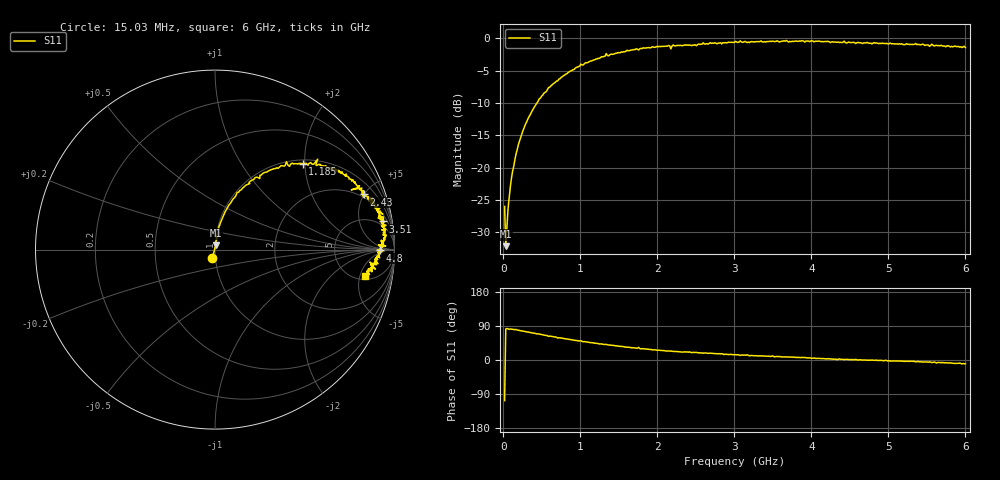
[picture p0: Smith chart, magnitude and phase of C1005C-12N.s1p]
!	Network	Analyzer	HP8753E.07.74:	Oct	30	2002	Serial	No.	JP38451487
!	Hewlett-Packard
!	7	Sep	2009	8:43:02
!	Frequency	S11
#	HZ	S	RI	R	50
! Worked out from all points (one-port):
!   400 points, 15.03 MHz to 6 GHz, reference 50 ohm
!   lowest |S11| = -32.1 dB at 30.03 MHz (marker M1), VSWR 1.05, Z = 50.3 + j2.47 ohm
!   |S11| at or under -10 dB: start of sweep to 435.5 MHz
!   S11 on the Smith chart (normalised r, x): 15.03 MHz: 0.97, -0.09; 1.185 GHz: 1.09, +1.95; 2.43 GHz: 1.77, +4.97; 3.51 GHz: 4, +11; 4.8 GHz: 23, -1; 6 GHz: 5.85, -6.14
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1.502992e7  -0.0148 -0.048
3.002985e7  0.0036 0.0245
6.00297e7  0.00645 0.048
1.050295e8  0.0127 0.0827
1.650292e8  0.0214 0.127
2.550287e8  0.0469 0.189
4.650277e8  0.123 0.318
7.650262e8  0.27 0.427
1.005025e9  0.398 0.49
1.185024e9  0.488 0.478
1.335023e9  0.572 0.504
1.365023e9  0.564 0.466
1.515022e9  0.626 0.454
1.93502e9  0.77 0.387
2.145019e9  0.805 0.356
2.175019e9  0.759 0.333
2.205019e9  0.819 0.342
2.265019e9  0.818 0.332
2.430018e9  0.829 0.307
3.015015e9  0.918 0.23
3.510012e9  0.935 0.157
3.765011e9  0.935 0.129
4.335008e9  0.932 0.0158
4.365008e9  0.926 0.0487
4.515007e9  0.928 0.0215
4.800006e9  0.918 -0.00482
5.265004e9  0.897 -0.0555
6e9  0.838 -0.145
